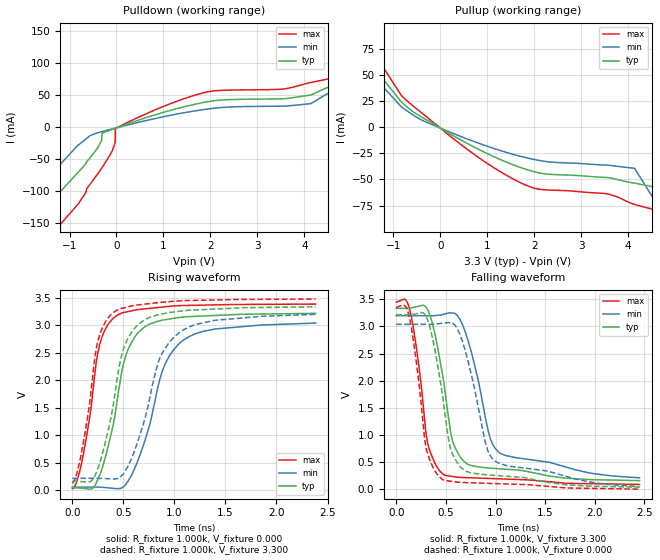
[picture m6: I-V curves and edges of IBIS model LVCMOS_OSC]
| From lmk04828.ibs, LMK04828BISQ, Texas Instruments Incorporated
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|   Model LVCMOS
[Model] LVCMOS_OSC
Model_type   Output
Polarity   Non-Inverting
Vmeas = 1.65
Vref = 1.65
Cref = 0pF
Rref = 50
|   typ   min   max
C_comp   2.0305p   1.9034p   2.088p
|   (nom PVT)   (slow PVT)   (fast PVT)
|C_comp (High state)   2.0305p   1.9034p   2.088p
|   (nom PVT)   (fast PVT)   (slow PVT)
|C_comp (Low state)   1.674p   1.576p   1.7125p
[Voltage Range]   3.3   3.15   3.45
[Temperature Range]   27   125   -40
[Pullup Reference]   3.3   3.15   3.45
[Pulldown Reference]   0   0   0
[Power Clamp Reference]   3.3   3.15   3.45
[GND Clamp Reference]   0   0   0
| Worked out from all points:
|   slope of the pulldown table from 0 to 0.495 V, typ, clamps not added: 39 ohm
|   slope of the pullup table from 0 to 0.495 V, typ, clamps not added: 39 ohm
|   falling waveform, R_fixture 1.000k, V_fixture 3.300: 20-80 % time 178ps typ, 232ps min, 141ps max; typ from 3.33 V to 0.161 V
|   rising waveform, R_fixture 1.000k, V_fixture 0.000: 20-80 % time 217ps typ, 286ps min, 165ps max; typ from 0.04 V to 3.22 V
|   rising waveform, R_fixture 1.000k, V_fixture 3.300: 20-80 % time 216ps typ, 290ps min, 164ps max; typ from 0.161 V to 3.33 V
|   falling waveform, R_fixture 1.000k, V_fixture 0.000: 20-80 % time 173ps typ, 228ps min, 136ps max; typ from 3.22 V to 0.04 V
[Pulldown]
|   Voltage   I(typ)   I(min)   I(max)
-3.3V     -785.5mA   -668.8mA   -867.2mA
-2.023V   -246.5mA   -189mA     -294.6mA
-1.795V   -190.1mA   -138.6mA   -222.1mA
-1.384V   -116.4mA   -73.03mA   -168.4mA
-270.6mV  -8.334mA   -6.174mA   -59.44mA
-28.05mV  -1.86mA    -1.561mA   -24.12mA
-23.1mV   -1.728mA   -1.467mA   -2.069mA
1.883V    39.05mA    27.81mA    54.38mA
4.14V     50.34mA    36.91mA    70.06mA
4.882V    75.33mA    69.76mA    81.21mA
5.857V    139.3mA    152.4mA    153.1mA
6.595V    236.7mA    234.9mA    258.1mA
[Pullup]
|   Voltage   I(typ)   I(min)   I(max)
-3.3V     231.3mA    210.5mA    276.4mA
-2.439V   117.7mA    114.3mA    148.6mA
-2.117V   95.35mA    82.53mA    119.7mA
-597.3mV  15.15mA    12.07mA    20.85mA
1.808V    -40.09mA   -29.02mA   -55.2mA
3.551V    -48.13mA   -36.34mA   -63.71mA
4.135V    -53.52mA   -39.28mA   -73.88mA
4.531V    -56.99mA   -67.68mA   -78.6mA
4.536V    -92.41mA   -68.19mA   -78.65mA
4.848V    -132.4mA   -102.4mA   -82.42mA
4.853V    -133.1mA   -103mA     -162.6mA
6.595V    -760.8mA   -664.5mA   -800.4mA
[Ramp]
R_load = 1000
|   typ   min   max
dV/dt_r   1.90033/2.16555e-10   1.77642/2.86485e-10   2.00968/1.6517e-10
dV/dt_f   1.9019/1.78168e-10   1.76631/2.32547e-10   2.01351/1.3979e-10
[Falling Waveform]
R_fixture = 1.000k
V_fixture = 3.300
V_fixture_min = 3.150
V_fixture_max = 3.450
C_fixture = 0.000
|  time   V(typ)   V(min)   V(max)
|   0.000S   3.335V   3.198V   3.447V
|  525.378ps   3.335V   3.197V   3.446V
|  570.226ps   3.335V   3.197V   3.461V
|  632.925ps   3.335V   3.197V   3.505V
|  644.789ps   3.335V   3.197V   3.493V
|  658.752ps   3.335V   3.197V   3.458V
|  674.533ps   3.335V   3.197V   3.388V
|  687.793ps   3.335V   3.197V   3.301V
|  688.844ps   3.335V   3.197V   3.292V
|  704.340ps   3.342V   3.197V   3.162V
|  720.028ps   3.349V   3.197V   3.007V
|  725.267ps   3.351V   3.197V   2.950V
|  748.087ps   3.361V   3.197V   2.679V
|  750.539ps   3.362V   3.197V   2.648V
|  752.831ps   3.363V   3.197V   2.619V
|  779.165ps   3.374V   3.197V   2.262V
|  801.432ps   3.384V   3.197V   1.932V
|  811.212ps   3.388V   3.197V   1.762V
|  820.801ps   3.392V   3.197V   1.579V
|  838.066ps   3.380V   3.197V   1.250V
|  845.309ps   3.366V   3.197V   1.112V
|  846.800ps   3.363V   3.197V   1.087V
|  853.492ps   3.350V   3.197V   989.591mV
|  857.798ps   3.341V   3.197V   942.739mV
|  862.378ps   3.326V   3.197V   892.893mV
|  868.349ps   3.305V   3.197V   842.258mV
|  874.444ps   3.284V   3.197V   798.306mV
|  875.406ps   3.279V   3.197V   791.369mV
|  894.414ps   3.183V   3.197V   679.201mV
|  896.701ps   3.171V   3.197V   669.201mV
|  915.261ps   3.052V   3.197V   588.048mV
|  921.617ps   3.007V   3.197V   560.254mV
|  921.619ps   3.007V   3.197V   560.247mV
|  940.277ps   2.858V   3.200V   478.666mV
|  944.882ps   2.822V   3.201V   463.684mV
|  962.211ps   2.665V   3.204V   407.309mV
|  965.968ps   2.631V   3.205V   397.240mV
|  969.807ps   2.595V   3.206V   386.950mV
|  982.111ps   2.469V   3.208V   353.974mV
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0s        3.335V     3.198V     3.447V
137.5ps   3.335V     3.197V     3.301V
312.1ps   3.326V     3.197V     892.9mV
471.7ps   2.056V     3.221V     279.8mV
552.7ps   1.01V      3.251V     241.1mV
626.7ps   651.2mV    3.173V     222.9mV
760.7ps   437.6mV    2.501V     212.6mV
946.7ps   390.3mV    941.2mV    200.2mV
1.031ns   379.6mV    687.2mV    194.6mV
2.45ns    160.7mV    212.9mV    90.81mV
[Rising Waveform]
R_fixture = 1.000k
V_fixture = 0.000
V_fixture_min = 0.000
V_fixture_max = 0.000
C_fixture = 0.000
|  time   V(typ)   V(min)   V(max)
|   0.000S   40.314mV   52.070mV   31.962mV
|  510.610ps   40.615mV   52.359mV   32.744mV
|  603.958ps   40.670mV   52.412mV   10.124mV
|  613.161ps   40.675mV   52.417mV   14.643mV
|  621.832ps   40.680mV   52.422mV   24.595mV
|  644.789ps   40.694mV   52.435mV   79.998mV
|  658.752ps   40.702mV   52.443mV   142.405mV
|  669.338ps   40.708mV   52.449mV   211.714mV
|  687.793ps   37.014mV   52.459mV   332.536mV
|  704.340ps   33.703mV   52.468mV   466.933mV
|  720.028ps   30.563mV   52.477mV   608.888mV
|  727.887ps   28.990mV   52.482mV   684.678mV
|  759.357ps   22.691mV   52.500mV   1.012V
|  761.163ps   22.330mV   52.501mV   1.032V
|  763.607ps   21.841mV   52.502mV   1.059V
|  766.480ps   21.266mV   52.504mV   1.090V
|  792.637ps   16.030mV   52.518mV   1.393V
|  793.783ps   15.801mV   52.519mV   1.409V
|  801.432ps   19.548mV   52.523mV   1.515V
|  805.769ps   21.673mV   52.526mV   1.587V
|  811.212ps   27.825mV   52.529mV   1.677V
|  820.801ps   38.663mV   52.534mV   1.843V
|  830.305ps   58.756mV   52.540mV   2.007V
|  838.066ps   75.165mV   52.544mV   2.128V
|  849.784ps   124.966mV   52.551mV   2.310V
|  853.492ps   140.725mV   52.553mV   2.358V
|  862.378ps   178.490mV   52.558mV   2.458V
|  884.127ps   270.920mV   52.570mV   2.643V
|  894.414ps   314.638mV   52.576mV   2.712V
|  896.337ps   322.811mV   52.577mV   2.723V
|  896.701ps   324.357mV   52.512mV   2.725V
|  906.974ps   384.282mV   50.677mV   2.784V
|  915.261ps   432.617mV   49.197mV   2.825V
|  921.619ps   472.402mV   48.062mV   2.857V
|  922.019ps   475.139mV   47.990mV   2.859V
|  957.140ps   715.143mV   41.718mV   2.986V
|  962.211ps   754.067mV   40.812mV   3.005V
|  968.844ps   804.986mV   39.628mV   3.023V
|  999.423ps   1.040V   34.167mV   3.090V
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0s        40.31mV    52.07mV    31.96mV
103.5ps   30.56mV    52.48mV    608.9mV
221.5ps   75.16mV    52.54mV    2.128V
290.4ps   384.3mV    50.68mV    2.784V
399.5ps   1.179V     31.21mV    3.126V
494.5ps   2.243V     50.53mV    3.227V
605.5ps   2.77V      372.4mV    3.272V
901.5ps   3.099V     2.262V     3.334V
1.089ns   3.15V      2.732V     3.358V
2.383ns   3.216V     3.039V     3.385V
[Rising Waveform]
R_fixture = 1.000k
V_fixture = 3.300
V_fixture_min = 3.150
V_fixture_max = 3.450
C_fixture = 0.000
|  time   V(typ)   V(min)   V(max)
|   0.000S   160.672mV   212.877mV   123.424mV
|  510.610ps   161.315mV   213.315mV   124.196mV
|  596.211ps   161.423mV   213.388mV   105.326mV
|  603.958ps   161.433mV   213.395mV   107.216mV
|  613.161ps   161.444mV   213.403mV   115.785mV
|  632.925ps   161.469mV   213.419mV   160.362mV
|  644.789ps   161.484mV   213.429mV   208.646mV
|  649.668ps   161.490mV   213.434mV   236.687mV
|  658.752ps   160.211mV   213.442mV   288.894mV
|  687.793ps   156.120mV   213.467mV   509.409mV
|  704.340ps   153.790mV   213.481mV   659.139mV
|  737.386ps   149.136mV   213.509mV   999.595mV
|  741.944ps   148.494mV   213.513mV   1.050V
|  745.427ps   148.004mV   213.516mV   1.089V
|  770.133ps   144.524mV   213.537mV   1.382V
|  780.045ps   145.408mV   213.546mV   1.500V
|  785.270ps   148.307mV   213.550mV   1.562V
|  792.637ps   152.394mV   213.556mV   1.671V
|  793.783ps   153.030mV   213.557mV   1.690V
|  820.801ps   199.091mV   213.581mV   2.153V
|  824.358ps   210.745mV   213.584mV   2.214V
|  838.066ps   255.655mV   213.596mV   2.417V
|  840.686ps   268.098mV   213.598mV   2.456V
|  845.309ps   290.048mV   213.602mV   2.512V
|  853.492ps   328.909mV   213.609mV   2.598V
|  868.349ps   399.459mV   213.622mV   2.720V
|  871.245ps   413.210mV   213.624mV   2.739V
|  874.444ps   428.403mV   213.378mV   2.761V
|  875.406ps   434.145mV   213.304mV   2.768V
|  884.127ps   486.191mV   212.634mV   2.821V
|  896.701ps   561.233mV   211.669mV   2.885V
|  906.974ps   629.866mV   210.880mV   2.937V
|  915.261ps   685.226mV   210.243mV   2.968V
|  934.335ps   823.580mV   208.779mV   3.039V
|  940.277ps   870.168mV   208.323mV   3.061V
|  962.211ps   1.042V   206.638mV   3.122V
|  965.968ps   1.072V   206.350mV   3.130V
|  969.807ps   1.103V   206.054mV   3.139V
|  974.070ps   1.138V   205.727mV   3.148V
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0s        160.7mV    212.9mV    123.4mV
120.8ps   149.1mV    213.5mV    999.6mV
221.5ps   255.7mV    213.6mV    2.417V
290.4ps   629.9mV    210.9mV    2.937V
399.5ps   1.527V     202.5mV    3.226V
475.5ps   2.396V     247mV      3.303V
581.5ps   2.875V     584.7mV    3.352V
859.5ps   3.197V     2.413V     3.415V
1.043ns   3.252V     2.86V      3.443V
2.383ns   3.335V     3.198V     3.476V
[Falling Waveform]
R_fixture = 1.000k
V_fixture = 0.000
V_fixture_min = 0.000
V_fixture_max = 0.000
C_fixture = 0.000
|  time   V(typ)   V(min)   V(max)
|   0.000S   3.216V   3.039V   3.352V
|  525.378ps   3.215V   3.039V   3.351V
|  570.226ps   3.215V   3.039V   3.365V
|  621.832ps   3.215V   3.039V   3.400V
|  644.789ps   3.215V   3.039V   3.375V
|  658.752ps   3.215V   3.039V   3.326V
|  669.338ps   3.215V   3.039V   3.263V
|  674.533ps   3.216V   3.039V   3.233V
|  687.793ps   3.218V   3.039V   3.124V
|  704.340ps   3.221V   3.039V   2.961V
|  725.267ps   3.224V   3.039V   2.717V
|  727.887ps   3.225V   3.039V   2.684V
|  729.146ps   3.225V   3.039V   2.668V
|  733.126ps   3.227V   3.039V   2.617V
|  754.448ps   3.236V   3.039V   2.323V
|  785.270ps   3.249V   3.039V   1.863V
|  792.637ps   3.252V   3.039V   1.743V
|  801.432ps   3.256V   3.039V   1.587V
|  805.769ps   3.257V   3.039V   1.504V
|  820.801ps   3.252V   3.039V   1.218V
|  830.305ps   3.238V   3.039V   1.037V
|  838.066ps   3.226V   3.039V   910.933mV
|  838.375ps   3.225V   3.039V   905.911mV
|  840.686ps   3.218V   3.039V   874.060mV
|  849.784ps   3.189V   3.039V   774.348mV
|  853.492ps   3.178V   3.039V   742.633mV
|  857.283ps   3.166V   3.039V   713.842mV
|  857.798ps   3.164V   3.039V   710.884mV
|  874.444ps   3.082V   3.039V   615.119mV
|  884.127ps   3.020V   3.039V   559.417mV
|  896.701ps   2.938V   3.039V   506.675mV
|  915.261ps   2.793V   3.039V   428.823mV
|  921.617ps   2.737V   3.039V   402.159mV
|  922.019ps   2.733V   3.039V   400.473mV
|  934.335ps   2.623V   3.042V   359.468mV
|  940.277ps   2.565V   3.043V   339.685mV
|  944.882ps   2.521V   3.044V   327.173mV
|  951.250ps   2.456V   3.045V   309.870mV
|  968.844ps   2.273V   3.049V   262.063mV
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0s        3.216V     3.039V     3.352V
137.5ps   3.218V     3.039V     3.124V
307ps     3.166V     3.039V     713.8mV
465.7ps   1.736V     3.06V      180.9mV
544.7ps   763.1mV    3.069V     150.4mV
615.7ps   488.6mV    2.955V     132.2mV
723.7ps   321.4mV    2.36V      123.6mV
900.7ps   269.1mV    839.8mV    112.5mV
996.7ps   256.4mV    517.3mV    106.5mV
2.45ns    40.31mV    52.07mV    3.732mV
